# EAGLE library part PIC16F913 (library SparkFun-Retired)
PIC16F913 IC PIC MCU FLASH 4KX14 28SOIC SparkFun Products Polar Heart Rate Monitor Interface (SEN-08661) Short timer
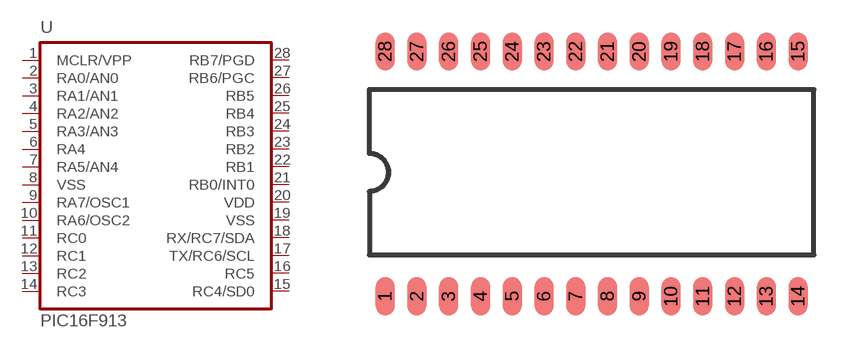
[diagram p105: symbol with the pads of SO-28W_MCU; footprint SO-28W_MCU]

Designator prefix -

## PIC16F913SOIC28  [SO-28W_MCU]
1  MCLR/VPP
2  RA0/AN0
3  RA1/AN1
4  RA2/AN2
5  RA3/AN3
6  RA4
7  RA5/AN4
8  VSS  pwr
9  RA7/OSC1
10  RA6/OSC2
11  RC0
12  RC1
13  RC2
14  RC3
15  RC4/SD0
16  RC5
17  TX/RC6/SCL
18  RX/RC7/SDA  in
19  VSS  pwr
20  VDD  pwr
21  RB0/INT0
22  RB1
23  RB2
24  RB3
25  RB4
26  RB5
27  RB6/PGC
28  RB7/PGD

## Footprint SO-28W_MCU (pad centres in mm)
Small Outline Wide Plastic Gull Wing 300-mil body, package type SO
smd 0.762 x 1.524: 1 -8.255,-4.953; 2 -6.985,-4.953; 3 -5.715,-4.953; 4 -4.445,-4.953; 5 -3.175,-4.953; 6 -1.905,-4.953; 7 -0.635,-4.953; 8 0.635,-4.953; 9 1.905,-4.953; 10 3.175,-4.953; 11 4.445,-4.953; 12 5.715,-4.953; 13 6.985,-4.953; 14 8.255,-4.953; 15 8.255,4.826; 16 6.985,4.826; 17 5.715,4.826; 18 4.445,4.826; 19 3.175,4.826; 20 1.905,4.826; 21 0.635,4.826; 22 -0.635,4.826; 23 -1.905,4.826; 24 -3.175,4.826; 25 -4.445,4.826; 26 -5.715,4.826; 27 -6.985,4.826; 28 -8.255,4.826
